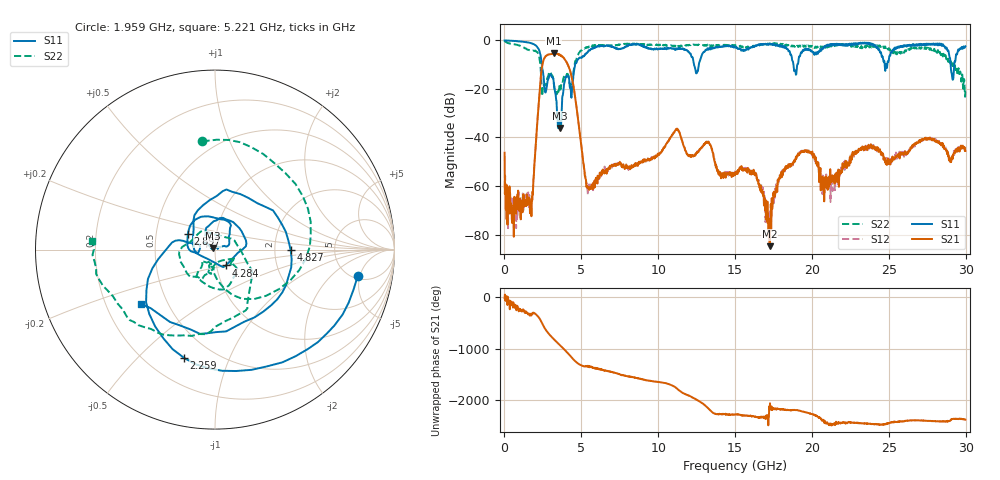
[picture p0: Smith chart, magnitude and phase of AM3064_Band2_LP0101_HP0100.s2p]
# Hz S DB R 50.0
!freq dBS11 angS11 dBS21 angS21 dBS12 angS12 dBS22 angS22
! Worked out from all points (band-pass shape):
!   1600 points, 10 MHz to 29.98 GHz, reference 50 ohm
!   highest |S21| = -5.34 dB at 3.215 GHz (marker M1); lowest = -84.8 dB at 17.25 GHz (marker M2)
!   |S21| within 3 dB of the highest: 2.532 GHz to 3.977 GHz (1.445 GHz wide, 44.4 % of centre)
!   lowest |S11| = -36.1 dB at 3.628 GHz (marker M3), VSWR 1.03, Z = 48.7 + j0.852 ohm
!   |S11| at or under -10 dB: 2.43 GHz to 4.595 GHz (2.164 GHz wide, 61.6 % of centre); 12.33 GHz to 12.64 GHz (314 MHz wide, 2.52 % of centre); 18.8 GHz to 19.05 GHz (251.6 MHz wide, 1.33 % of centre)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
!   |S22| runs from -23.3 to -0.2 dB; largest |S21 - S12| = 0.015
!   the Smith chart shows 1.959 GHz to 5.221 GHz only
!   S11 on the Smith chart (normalised r, x): 1.959 GHz: 5.50, -4.62; 2.259 GHz: 0.35, -0.69; 2.897 GHz: 0.73, +0.13; 4.284 GHz: 1.11, -0.20; 4.827 GHz: 2.46, -0.02; 5.221 GHz: 0.36, -0.29
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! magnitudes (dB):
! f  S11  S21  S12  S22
! 10 MHz  0.0  -46.3  -61.0  -0.2
! 628.5 MHz  -0.2  -68.2  -72.1  -1.6
! 1.697 GHz  -1.1  -67.1  -66.3  -4.2
! 1.959 GHz  -1.8  -50.1  -50.4  -4.3
! 2.259 GHz  -4.0  -23.2  -23.2  -6.9
! 2.897 GHz  -15.2  -5.8  -5.7  -13.4
! 3.215 GHz  -17.6  -5.3  -5.4  -18.0
! 3.628 GHz  -36.1  -6.1  -6.1  -19.9
! 4.284 GHz  -19.4  -12.9  -12.8  -18.0
! 4.827 GHz  -7.5  -34.3  -34.3  -5.4
! 5.015 GHz  -7.3  -44.1  -44.1  -4.1
! 5.221 GHz  -5.8  -55.6  -54.4  -3.3
! 10 GHz  -3.5  -46.6  -46.9  -1.9
! 11.22 GHz  -3.7  -36.4  -36.4  -2.2
! 15 GHz  -2.7  -55.4  -54.6  -2.0
! 16.26 GHz  -2.4  -54.6  -54.7  -2.6
! 17.25 GHz  -1.5  -84.8  -74.6  -1.2
! 18.12 GHz  -2.9  -54.8  -53.7  -1.6
! 19.99 GHz  -4.4  -46.8  -46.4  -2.2
! 20.87 GHz  -2.3  -57.0  -59.3  -3.0
! 25 GHz  -8.3  -49.7  -49.9  -3.2
! 29.98 GHz  -2.4  -45.5  -45.7  -20.2
